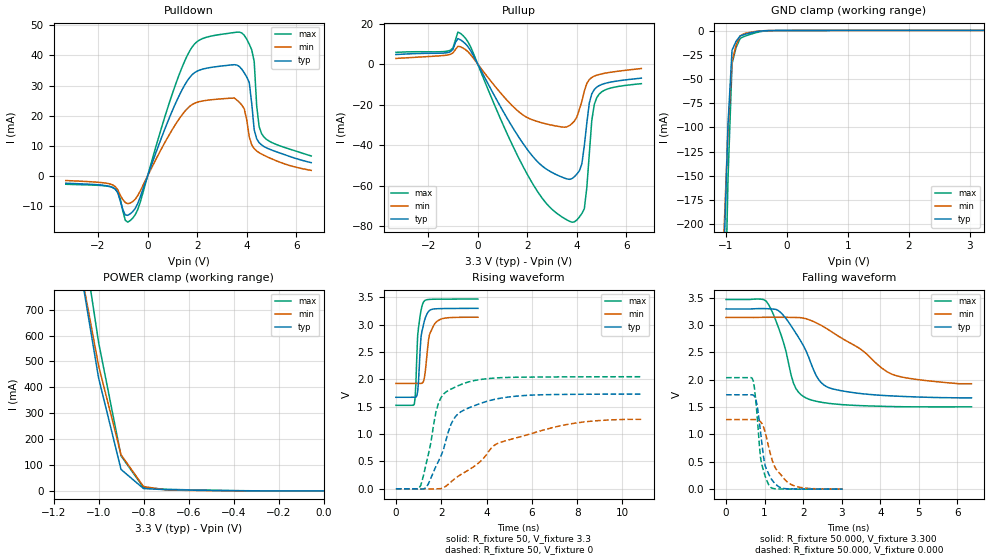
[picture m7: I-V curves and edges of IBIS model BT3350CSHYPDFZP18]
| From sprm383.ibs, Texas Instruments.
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|   Model Cell BT3350CSHYPDFZP18
[Model]   BT3350CSHYPDFZP18
Model_type   I/O
Polarity   Non-Inverting
Enable   Active-Low
Vinl =  0.8V
Vinh =  2V
Cref =  15.0000pF
Rref =  100.0000M
Vref =  0V
Vmeas =  1.65
C_comp   1.740586p   1.693574p   1.782556p
[Model Spec]
Vinl   0.8V   0.8V   0.8V
Vinh   2V   2V   2V
[Temperature Range]   25   105   0
[Voltage Range]   3.3   3.14   3.47
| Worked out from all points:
|   slope of the pulldown table from 0 to 0.495 V, typ, clamps not added: 44 ohm
|   slope of the pullup table from 0 to 0.495 V, typ, clamps not added: 42.8 ohm
|   GND clamp passes 1 mA (typ) near -0.49 V on its own axis
|   POWER clamp passes 1 mA (typ) near -0.40 V on its own axis
|   rising waveform, R_fixture 50, V_fixture 3.3: 20-80 % time 201ps typ, 262ps min, 162ps max; typ from 1.67 V to 3.3 V
|   rising waveform, R_fixture 50, V_fixture 0: 20-80 % time 1.09ns typ, 3.19ns min, 650ps max; typ from 0 V to 1.73 V
|   falling waveform, R_fixture 50.000, V_fixture 3.300: 20-80 % time 709ps typ, 1.43ns min, 479ps max; typ from 3.29 V to 1.67 V
|   falling waveform, R_fixture 50.000, V_fixture 0.000: 20-80 % time 225ps typ, 408ps min, 175ps max; typ from 1.73 V to 0.001 V
[POWER_clamp]
|   voltage   I(typ)   I(min)   I(max)
-3.3V     15.06A     13.76A     16A
-1.067V   785.8mA    796.6mA    959.4mA
-1.033V   611.7mA    640.9mA    767.4mA
-1V       437.6mA    485.1mA    575.3mA
-900mV    83.19mA    139.9mA    135.7mA
-800mV    9.173mA    17.09mA    12.71mA
-700mV    4.913mA    3.842mA    6.411mA
-400mV    992.1uA    528.5uA    1.341mA
-11.55fV  142.7uA    86.75uA    197.1uA
[Pulldown]
|   voltage   I(typ)   I(min)   I(max)
-3.3V     -2.42mA    -1.536mA   -2.768mA
-1.4V     -3.865mA   -3.029mA   -3.892mA
-700mV    -12.57mA   -9.01mA    -14.79mA
1.7V      32.7mA     23.11mA    41.52mA
3.6V      36.8mA     25.18mA    47.71mA
3.9V      34.21mA    22.24mA    46.65mA
4.1V      30.98mA    12.94mA    43.73mA
4.2V      24.06mA    10.3mA     41.84mA
4.3V      15.3mA     9.054mA    37.97mA
4.4V      12.31mA    8.283mA    23.22mA
4.6V      10.26mA    7.234mA    13.99mA
6.6V      4.412mA    1.834mA    6.626mA
[Pullup]
|   voltage   I(typ)   I(min)   I(max)
-3.3V     4.71mA     2.781mA    5.78mA
-1.2V     5.694mA    4.518mA    6.444mA
-800mV    12.56mA    8.755mA    15.79mA
-600mV    11.14mA    7.956mA    14.14mA
2.2V      -45.34mA   -27.51mA   -58.77mA
3.8V      -56.58mA   -29.42mA   -78.12mA
4.1V      -52.76mA   -22.36mA   -75.56mA
4.3V      -40.26mA   -13.34mA   -71.48mA
4.4V      -29.2mA    -9.578mA   -61.01mA
4.6V      -14.75mA   -6.625mA   -27.92mA
4.8V      -11.42mA   -5.502mA   -16.63mA
6.6V      -6.965mA   -2.214mA   -9.682mA
[GND_clamp]
|   voltage   I(typ)   I(min)   I(max)
-3.3V     -17.31A    -15.81A    -18.25A
-1.033V   -232.2mA   -209.7mA   -350mA
-966.7mV  -97.23mA   -102.7mA   -153.5mA
-900mV    -20.27mA   -31.82mA   -34.24mA
-833.3mV  -11.04mA   -15mA      -17.47mA
-766.7mV  -5.659mA   -5.47mA    -8.107mA
-700mV    -4.122mA   -3.24mA    -6.148mA
-500mV    -1.111mA   -790.6uA   -2.074mA
-300mV    -91.74uA   -71.4uA    -180uA
3.233V    142.6uA    88.12uA    196.8uA
[Ramp]
| variable   typ   min   max
dV/dt_f   1.003771/0.713032n   0.7884886/1.610103n   1.181978/0.4787008n
dV/dt_r   1.045735/1.105045n   0.784976/3.396821n   1.233673/0.6480172n
R_load = 50
[Rising Waveform]
R_fixture = 50
V_fixture = 3.3
V_fixture_min = 3.14
V_fixture_max = 3.47
|   time   V(typ)   V(min)   V(max)
0s        1.671V     1.924V     1.525V
812ps     1.672V     1.925V     1.547V
848ps     1.672V     1.925V     1.659V
884ps     1.674V     1.925V     1.948V
960ps     1.776V     1.925V     2.8V
1.108ns   2.776V     1.925V     3.257V
1.22ns    3.005V     1.968V     3.412V
1.476ns   3.254V     2.805V     3.46V
1.736ns   3.287V     3.026V     3.463V
3.62ns    3.296V     3.134V     3.466V
[Rising Waveform]
R_fixture = 50
V_fixture = 0
V_fixture_min = 0
V_fixture_max = 0
|   time   V(typ)   V(min)   V(max)
0s        47.1uV     22.62uV    79.08uV
1.1ns     -7.278mV   -24.43uV   65.61mV
1.324ns   17.13mV    -1.638mV   437.9mV
1.764ns   407.6mV    -1.504mV   1.397V
1.876ns   500.8mV    -13.03uV   1.56V
2.428ns   1.174V     123.9mV    1.82V
2.648ns   1.328V     199.3mV    1.864V
4.748ns   1.663V     865.8mV    2.032V
7.844ns   1.725V     1.195V     2.045V
10.84ns   1.73V      1.269V     2.047V
[Falling Waveform]
R_fixture = 50.000
V_fixture = 3.300
V_fixture_min = 3.140
V_fixture_max = 3.470
|  time   V(typ)   V(min)   V(max)
0s        3.293V     3.138V     3.466V
1.036ns   3.299V     3.141V     3.439V
1.428ns   3.221V     3.141V     2.816V
1.752ns   2.914V     3.138V     1.93V
1.88ns    2.773V     3.136V     1.771V
2.144ns   2.41V      3.098V     1.645V
2.404ns   1.999V     3.017V     1.597V
2.792ns   1.828V     2.851V     1.558V
4.352ns   1.702V     2.088V     1.509V
6.364ns   1.669V     1.927V     1.505V
[Falling Waveform]
R_fixture = 50.000
V_fixture = 0.000
V_fixture_min = 0.000
V_fixture_max = 0.000
|  time   V(typ)   V(min)   V(max)
0s        1.725V     1.272V     2.038V
644ps     1.725V     1.272V     2.039V
708ps     1.718V     1.272V     1.973V
800ps     1.554V     1.27V      1.397V
892ps     1.061V     1.235V     588.8mV
1.016ns   427.3mV    1.036V     234.7mV
1.14ns    228.6mV    671.6mV    46.77mV
1.292ns   87.32mV    373.2mV    6.271mV
1.696ns   4.73mV     82.13mV    1.773mV
3.028ns   1.196mV    3.183mV    243.4uV
